FUNCTION "CENTR. 6  LATERALE SX" : VOID
TITLE =
VERSION : 0.1

BEGIN
NETWORK
TITLE =LETTURA STATUS WORD DA DRIVE
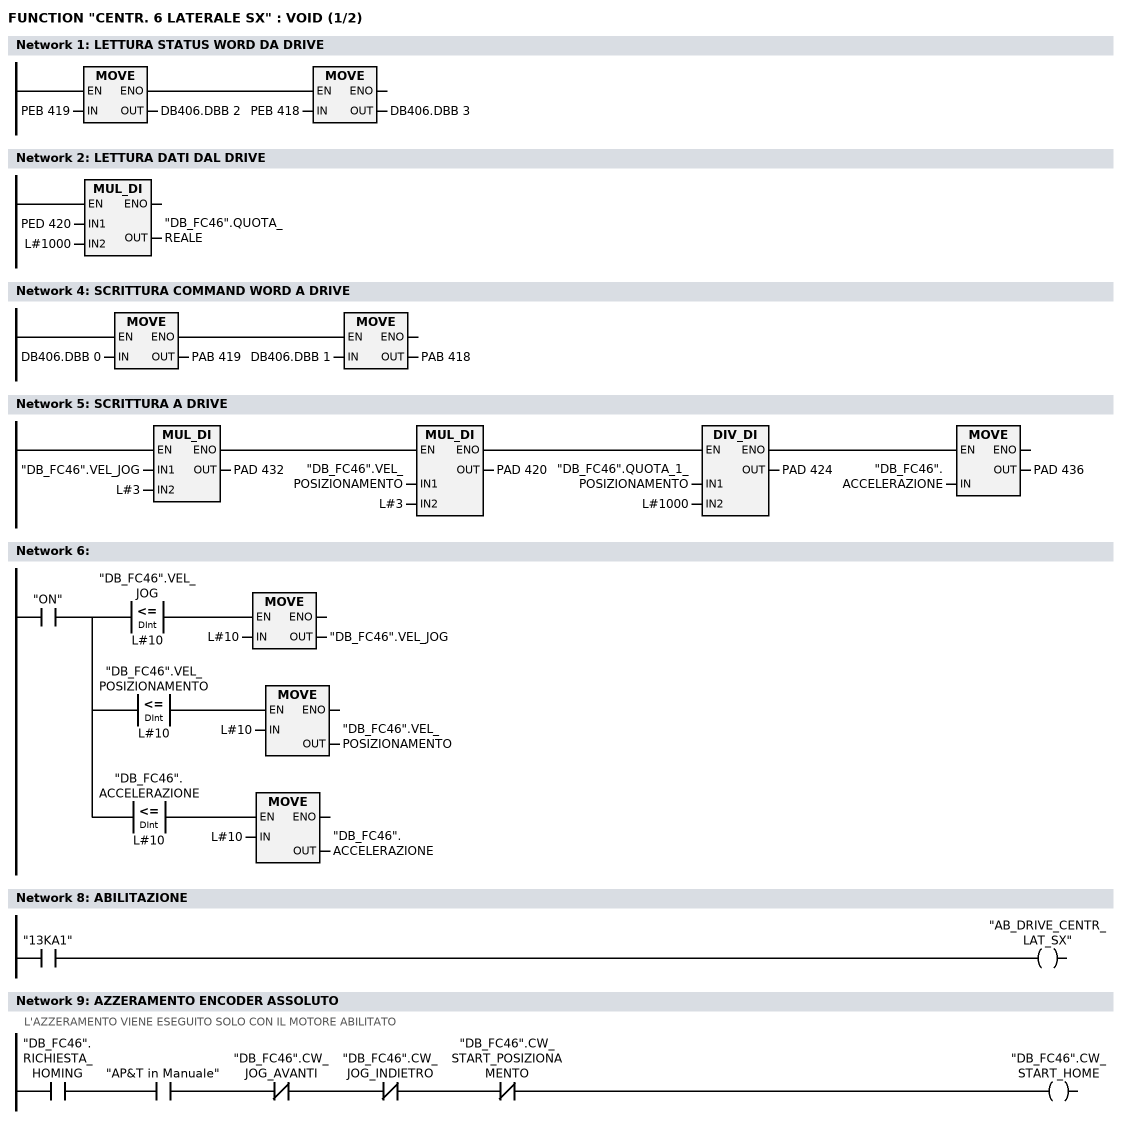
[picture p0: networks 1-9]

      U(    ;
      L     PEB  419;
      T     DB406.DBB    2;
      SET   ;
      SAVE  ;
      CLR   ;
      U     BIE;
      )     ;
      SPBNB _001;
      L     PEB  418;
      T     DB406.DBB    3;
_001: NOP   0;
NETWORK
TITLE =LETTURA DATI DAL DRIVE

      L     PED  420;
      L     L#1000;
      *D    ;
      T     "DB_FC46".QUOTA_REALE;
      NOP   0;
NETWORK
TITLE =

NETWORK
TITLE =SCRITTURA COMMAND WORD A DRIVE

      U(    ;
      L     DB406.DBB    0;
      T     PAB  419;
      SET   ;
      SAVE  ;
      CLR   ;
      U     BIE;
      )     ;
      SPBNB _002;
      L     DB406.DBB    1;
      T     PAB  418;
_002: NOP   0;
NETWORK
TITLE =SCRITTURA A DRIVE

      U(    ;
      U(    ;
      U(    ;
      L     "DB_FC46".VEL_JOG;
      L     L#3;
      *D    ;
      T     PAD  432;
      UN    OV;
      SAVE  ;
      CLR   ;
      U     BIE;
      )     ;
      SPBNB _003;
      L     "DB_FC46".VEL_POSIZIONAMENTO;
      L     L#3;
      *D    ;
      T     PAD  420;
      UN    OV;
      SAVE  ;
      CLR   ;
_003: U     BIE;
      )     ;
      SPBNB _004;
      L     "DB_FC46".QUOTA_1_POSIZIONAMENTO;
      L     L#1000;
      /D    ;
      T     PAD  424;
      UN    OV;
      SAVE  ;
      CLR   ;
_004: U     BIE;
      )     ;
      SPBNB _005;
      L     "DB_FC46".ACCELERAZIONE;
      T     PAD  436;
_005: NOP   0;
NETWORK
TITLE =

      U     "ON";
      =     L      0.0;
      U     L      0.0;
      U(    ;
      L     "DB_FC46".VEL_JOG;
      L     L#10;
      <=D   ;
      )     ;
      SPBNB _006;
      L     L#10;
      T     "DB_FC46".VEL_JOG;
_006: NOP   0;
      U     L      0.0;
      U(    ;
      L     "DB_FC46".VEL_POSIZIONAMENTO;
      L     L#10;
      <=D   ;
      )     ;
      SPBNB _007;
      L     L#10;
      T     "DB_FC46".VEL_POSIZIONAMENTO;
_007: NOP   0;
      U     L      0.0;
      U(    ;
      L     "DB_FC46".ACCELERAZIONE;
      L     L#10;
      <=D   ;
      )     ;
      SPBNB _008;
      L     L#10;
      T     "DB_FC46".ACCELERAZIONE;
_008: NOP   0;
NETWORK
TITLE =

NETWORK
TITLE =ABILITAZIONE

      U     "13KA1";
      =     "AB_DRIVE_CENTR_LAT_SX";
NETWORK
TITLE =AZZERAMENTO ENCODER ASSOLUTO
//L'AZZERAMENTO VIENE ESEGUITO SOLO CON IL MOTORE ABILITATO
      U     "DB_FC46".RICHIESTA_HOMING;
      U     "AP&T in Manuale";
      UN    "DB_FC46".CW_JOG_AVANTI;
      UN    "DB_FC46".CW_JOG_INDIETRO;
      UN    "DB_FC46".CW_START_POSIZIONAMENTO;
      =     "DB_FC46".CW_START_HOME;
NETWORK
TITLE =COMANDI DI JOG
//N.B. VERIFICARE QUOTE EXTRACORSA SOFTWARE
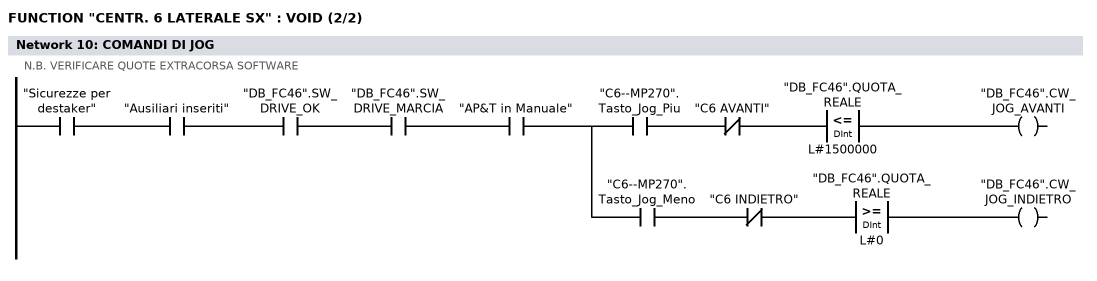
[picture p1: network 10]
      U     "Sicurezze per destaker";
      U     "Ausiliari inseriti";
      U     "DB_FC46".SW_DRIVE_OK;
      U     "DB_FC46".SW_DRIVE_MARCIA;
      U     "AP&T in Manuale";
      =     L      0.0;
      U     L      0.0;
      U     "C6--MP270".Tasto_Jog_Piu;
      UN    "C6 AVANTI";
      U(    ;
      L     "DB_FC46".QUOTA_REALE;
      L     L#1500000;
      <=D   ;
      )     ;
      =     "DB_FC46".CW_JOG_AVANTI;
      U     L      0.0;
      U     "C6--MP270".Tasto_Jog_Meno;
      UN    "C6 INDIETRO";
      U(    ;
      L     "DB_FC46".QUOTA_REALE;
      L     L#0;
      >=D   ;
      )     ;
      =     "DB_FC46".CW_JOG_INDIETRO;
NETWORK
TITLE =Centratore 6: Posizioni

      U     "ON";
      =     L      0.0;
      U     L      0.0;
      U(    ;
      L     "DB_FC46".QUOTA_REALE;
      L     L#100;
      <=D   ;
      )     ;
      U(    ;
      L     "DB_FC46".QUOTA_REALE;
      L     L#-100;
      >=D   ;
      )     ;
      =     "C6: Asse in pos.0";
      U(    ;
      U(    ;
      U     L      0.0;
      SPBNB _009;
      L     "MATRICOLA ATTUALE".C6_Posizione_1;
      L     L#100;
      -D    ;
      T     "CONFRONTI CENTRATORI".C6_Pos_1_Min;
      UN    OV;
      SAVE  ;
      CLR   ;
_009: U     BIE;
      )     ;
      SPBNB _00a;
      L     "MATRICOLA ATTUALE".C6_Posizione_1;
      L     L#200;
      +D    ;
      T     "CONFRONTI CENTRATORI".C6_Pos_1_Max;
      UN    OV;
      SAVE  ;
      CLR   ;
_00a: U     BIE;
      )     ;
      U(    ;
      L     "DB_FC46".QUOTA_REALE;
      L     "CONFRONTI CENTRATORI".C6_Pos_1_Min;
      >=D   ;
      )     ;
      U(    ;
      L     "DB_FC46".QUOTA_REALE;
      L     "CONFRONTI CENTRATORI".C6_Pos_1_Max;
      <=D   ;
      )     ;
      =     "C6: Asse in pos.1";
      U(    ;
      U(    ;
      U     L      0.0;
      SPBNB _00b;
      L     "MATRICOLA ATTUALE".C6_Posizione_2;
      L     L#100;
      -D    ;
      T     "CONFRONTI CENTRATORI".C6_Pos_2_Min;
      UN    OV;
      SAVE  ;
      CLR   ;
_00b: U     BIE;
      )     ;
      SPBNB _00c;
      L     "MATRICOLA ATTUALE".C6_Posizione_2;
      L     L#50000;
      +D    ;
      T     "CONFRONTI CENTRATORI".C6_Pos_2_Max;
      UN    OV;
      SAVE  ;
      CLR   ;
_00c: U     BIE;
      )     ;
      U(    ;
      L     "DB_FC46".QUOTA_REALE;
      L     "CONFRONTI CENTRATORI".C6_Pos_2_Min;
      >=D   ;
      )     ;
      UN    "C6: Asse in pos.3";
      UN    "C6: Asse in pos.4";
      =     "C6: Asse in pos.2";
      U(    ;
      U(    ;
      U     L      0.0;
      SPBNB _00d;
      L     "MATRICOLA ATTUALE".C6_Posizione_3;
      L     L#100;
      -D    ;
      T     "CONFRONTI CENTRATORI".C6_Pos_3_Min;
      UN    OV;
      SAVE  ;
      CLR   ;
_00d: U     BIE;
      )     ;
      SPBNB _00e;
      L     "MATRICOLA ATTUALE".C6_Posizione_3;
      L     L#50000;
      +D    ;
      T     "CONFRONTI CENTRATORI".C6_Pos_3_Max;
      UN    OV;
      SAVE  ;
      CLR   ;
_00e: U     BIE;
      )     ;
      U(    ;
      L     "DB_FC46".QUOTA_REALE;
      L     "CONFRONTI CENTRATORI".C6_Pos_3_Min;
      >=D   ;
      )     ;
      UN    "C6: Asse in pos.4";
      =     "C6: Asse in pos.3";
      U(    ;
      U(    ;
      U     L      0.0;
      SPBNB _00f;
      L     "MATRICOLA ATTUALE".C6_Posizione_4;
      L     L#100;
      -D    ;
      T     "CONFRONTI CENTRATORI".C6_Pos_4_Min;
      UN    OV;
      SAVE  ;
      CLR   ;
_00f: U     BIE;
      )     ;
      SPBNB _010;
      L     "MATRICOLA ATTUALE".C6_Posizione_4;
      L     L#100;
      +D    ;
      T     "CONFRONTI CENTRATORI".C6_Pos_4_Max;
      UN    OV;
      SAVE  ;
      CLR   ;
_010: U     BIE;
      )     ;
      U(    ;
      L     "DB_FC46".QUOTA_REALE;
      L     "CONFRONTI CENTRATORI".C6_Pos_4_Min;
      >=D   ;
      )     ;
      U(    ;
      L     "DB_FC46".QUOTA_REALE;
      L     "CONFRONTI CENTRATORI".C6_Pos_4_Max;
      <=D   ;
      )     ;
      =     "C6: Asse in pos.4";
NETWORK
TITLE =Centratore 6: consenso abilitazione passi
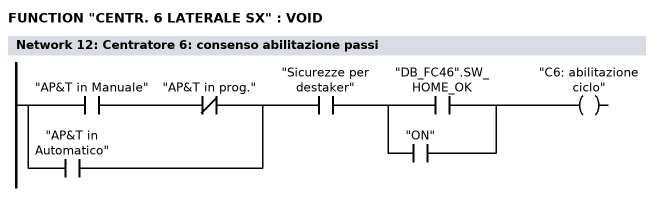
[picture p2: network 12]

      U(    ;
      U     "AP&T in Manuale";
      UN    "AP&T in prog.";
      O     "AP&T in Automatico";
      )     ;
      U     "Sicurezze per destaker";
      U(    ;
      O     "DB_FC46".SW_HOME_OK;
      O     "ON";
      )     ;
      =     "C6: abilitazione ciclo";
NETWORK
TITLE =Centratore 6: comando avvicinamento  (centraggi aperti)

      U(    ;
      U(    ;
      O     "Comando apre centraggi";
      O     "C6--MP270".Tasto_Indietro;
      O     ;
      U     "Apertura centratori";
      U(    ;
      O     "Centratori a riposo";
      O     "Centratori tutti chiusi";
      )     ;
      )     ;
      UN    "C6: Asse in pos.1";
      UN    "C6: comando arrivo";
      UN    "C6: comando a riposo";
      U     "C6: abilitazione ciclo";
      L     S5T#100MS;
      SE    T    197;
      NOP   0;
      NOP   0;
      NOP   0;
      U     T    197;
      )     ;
      S     "C6: comando avvicinam";
      U(    ;
      O     "C6: Asse in pos.1";
      O(    ;
      U(    ;
      O     "Ripristino centratori";
      O     "Comando riposo centraggi";
      O     "C6--MP270".Tasto_Riposo;
      )     ;
      FP    "C6: one shot 1";
      )     ;
      )     ;
      R     "C6: comando avvicinam";
      NOP   0;
NETWORK
TITLE =Centratore 6: comando arrivo (centraggi chiusi)

      U(    ;
      U(    ;
      O     "Comando chiude centraggi";
      O     "C6--MP270".Tasto_Avanti;
      O     ;
      U     "Chiusura centratori";
      U(    ;
      O     "Centratori tutti aperti";
      O     "Centratori a riposo";
      )     ;
      )     ;
      UN    "C6: Asse in pos.4";
      UN    "C6: comando avvicinam";
      UN    "C6: comando a riposo";
      U     "C6: abilitazione ciclo";
      L     S5T#100MS;
      SE    T    198;
      NOP   0;
      NOP   0;
      NOP   0;
      U     T    198;
      )     ;
      S     "C6: comando arrivo";
      U(    ;
      O     "C6: Asse in pos.4";
      O(    ;
      U(    ;
      O     "Ripristino centratori";
      O     "Comando riposo centraggi";
      O     "C6--MP270".Tasto_Riposo;
      )     ;
      FP    "C6: one shot 2";
      )     ;
      )     ;
      R     "C6: comando arrivo";
      NOP   0;
NETWORK
TITLE =Centratore 6: comando automatico centraggi a riposo

      U(    ;
      U(    ;
      O     "Comando riposo centraggi";
      O     "C6--MP270".Tasto_Riposo;
      )     ;
      UN    "C6: Asse in pos.0";
      UN    "C6: comando avvicinam";
      UN    "C6: comando arrivo";
      U     "C6: abilitazione ciclo";
      L     S5T#100MS;
      SE    T    199;
      NOP   0;
      NOP   0;
      NOP   0;
      U     T    199;
      )     ;
      S     "C6: comando a riposo";
      U(    ;
      O     "C6: Asse in pos.0";
      O(    ;
      U     "Ripristino centratori";
      FP    "C6: one shot 3";
      )     ;
      )     ;
      R     "C6: comando a riposo";
      NOP   0;
NETWORK
TITLE =Centratore 6: quote impostate per posizioni

      U     "ON";
      =     L      0.0;
      U(    ;
      U(    ;
      U     L      0.0;
      U     "C6: comando a riposo";
      UN    "C6: Asse in pos.0";
      SPBNB _011;
      L     0;
      T     "DB_FC46".QUOTA_1_POSIZIONAMENTO;
      SET   ;
      SAVE  ;
      CLR   ;
_011: U     BIE;
      )     ;
      SPBNB _012;
      L     L#150;
      T     "DB_FC46".VEL_POSIZIONAMENTO;
      SET   ;
      SAVE  ;
      CLR   ;
_012: U     BIE;
      )     ;
      SPBNB _013;
      L     L#1000;
      T     "DB_FC46".ACCELERAZIONE;
      SET   ;
      SAVE  ;
      CLR   ;
_013: U     BIE;
      =     "C6: Quote pronte pos.0";
      U(    ;
      U(    ;
      U     L      0.0;
      U     "C6: comando avvicinam";
      UN    "C6: Asse in pos.1";
      SPBNB _014;
      L     "MATRICOLA ATTUALE".C6_Posizione_1;
      T     "DB_FC46".QUOTA_1_POSIZIONAMENTO;
      SET   ;
      SAVE  ;
      CLR   ;
_014: U     BIE;
      )     ;
      SPBNB _015;
      L     "MATRICOLA ATTUALE".C6_Velocita_1;
      T     "DB_FC46".VEL_POSIZIONAMENTO;
      SET   ;
      SAVE  ;
      CLR   ;
_015: U     BIE;
      )     ;
      SPBNB _016;
      L     "MATRICOLA ATTUALE".C6_Accell_1;
      T     "DB_FC46".ACCELERAZIONE;
      SET   ;
      SAVE  ;
      CLR   ;
_016: U     BIE;
      =     "C6: Quote pronte pos.1";
      U     L      0.0;
      U     "C6: comando arrivo";
      =     L      0.1;
      U(    ;
      U(    ;
      U     L      0.1;
      UN    "C6: Asse in pos.2";
      SPBNB _017;
      L     "MATRICOLA ATTUALE".C6_Posizione_4;
      T     "DB_FC46".QUOTA_1_POSIZIONAMENTO;
      SET   ;
      SAVE  ;
      CLR   ;
_017: U     BIE;
      )     ;
      SPBNB _018;
      L     "MATRICOLA ATTUALE".C6_Velocita_2;
      T     "DB_FC46".VEL_POSIZIONAMENTO;
      SET   ;
      SAVE  ;
      CLR   ;
_018: U     BIE;
      )     ;
      SPBNB _019;
      L     "MATRICOLA ATTUALE".C6_Accell_2;
      T     "DB_FC46".ACCELERAZIONE;
      SET   ;
      SAVE  ;
      CLR   ;
_019: U     BIE;
      S     "C6: Quote pronte pos.2";
      U     L      0.1;
      U     "C6: Quote pronte pos.2";
      UN    "C6: Reset start pos.2";
      L     S5T#1S;
      SE    "C6: ritardo P2";
      NOP   0;
      NOP   0;
      NOP   0;
      U     "C6: ritardo P2";
      S     "C6: Reset start pos.2";
      R     "C6: Quote pronte pos.2";
      U     L      0.0;
      U     "C6: comando arrivo";
      =     L      0.1;
      U(    ;
      U(    ;
      U(    ;
      U     L      0.1;
      U     "C6: Asse in pos.2";
      UN    "C6: Asse in pos.3";
      SPBNB _01a;
      L     "MATRICOLA ATTUALE".C6_Posizione_4;
      T     "DB_FC46".QUOTA_1_POSIZIONAMENTO;
      SET   ;
      SAVE  ;
      CLR   ;
_01a: U     BIE;
      )     ;
      SPBNB _01b;
      L     "MATRICOLA ATTUALE".C6_Velocita_3;
      T     "DB_FC46".VEL_POSIZIONAMENTO;
      SET   ;
      SAVE  ;
      CLR   ;
_01b: U     BIE;
      )     ;
      SPBNB _01c;
      L     "MATRICOLA ATTUALE".C6_Accell_3;
      T     "DB_FC46".ACCELERAZIONE;
      SET   ;
      SAVE  ;
      CLR   ;
_01c: U     BIE;
      )     ;
      U     "C6: Reset start pos.2";
      S     "C6: Quote pronte pos.3";
      R     "C6: Reset start pos.2";
      U     L      0.1;
      U     "C6: Quote pronte pos.3";
      L     S5T#500MS;
      SE    "C6: ritardo P3";
      NOP   0;
      NOP   0;
      NOP   0;
      U     "C6: ritardo P3";
      S     "C6: Reset start pos.3";
      R     "C6: Quote pronte pos.3";
      U     L      0.0;
      U     "C6: comando arrivo";
      =     L      0.1;
      U(    ;
      U(    ;
      U(    ;
      U     L      0.1;
      U     "C6: Asse in pos.3";
      UN    "C6: Asse in pos.4";
      SPBNB _01d;
      L     "MATRICOLA ATTUALE".C6_Posizione_4;
      T     "DB_FC46".QUOTA_1_POSIZIONAMENTO;
      SET   ;
      SAVE  ;
      CLR   ;
_01d: U     BIE;
      )     ;
      SPBNB _01e;
      L     "MATRICOLA ATTUALE".C6_Velocita_4;
      T     "DB_FC46".VEL_POSIZIONAMENTO;
      SET   ;
      SAVE  ;
      CLR   ;
_01e: U     BIE;
      )     ;
      SPBNB _01f;
      L     "MATRICOLA ATTUALE".C6_Accell_4;
      T     "DB_FC46".ACCELERAZIONE;
      SET   ;
      SAVE  ;
      CLR   ;
_01f: U     BIE;
      )     ;
      U     "C6: Reset start pos.3";
      S     "C6: Quote pronte pos.4";
      R     "C6: Reset start pos.3";
      U     L      0.1;
      U     "C6: Quote pronte pos.4";
      L     S5T#500MS;
      SE    "C6: ritardo P4";
      NOP   0;
      NOP   0;
      NOP   0;
      U     "C6: ritardo P4";
      S     "C6: Reset start pos.4";
      R     "C6: Quote pronte pos.4";
NETWORK
TITLE =Centratore 6: reset impostate
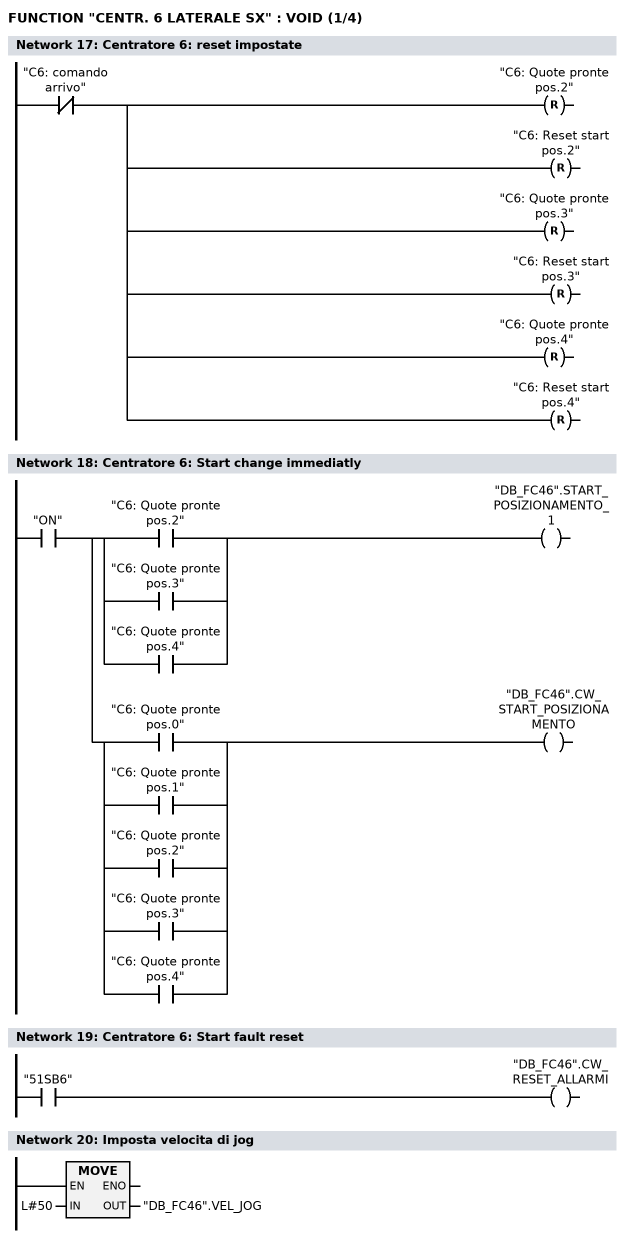
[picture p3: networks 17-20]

      UN    "C6: comando arrivo";
      R     "C6: Quote pronte pos.2";
      R     "C6: Reset start pos.2";
      R     "C6: Quote pronte pos.3";
      R     "C6: Reset start pos.3";
      R     "C6: Quote pronte pos.4";
      R     "C6: Reset start pos.4";
NETWORK
TITLE =Centratore 6: Start change immediatly

      U     "ON";
      =     L      0.0;
      U     L      0.0;
      U(    ;
      O     "C6: Quote pronte pos.2";
      O     "C6: Quote pronte pos.3";
      O     "C6: Quote pronte pos.4";
      )     ;
      =     "DB_FC46".START_POSIZIONAMENTO_1;
      U     L      0.0;
      U(    ;
      O     "C6: Quote pronte pos.0";
      O     "C6: Quote pronte pos.1";
      O     "C6: Quote pronte pos.2";
      O     "C6: Quote pronte pos.3";
      O     "C6: Quote pronte pos.4";
      )     ;
      =     "DB_FC46".CW_START_POSIZIONAMENTO;
NETWORK
TITLE =Centratore 6: Start fault reset

      U     "51SB6";
      =     "DB_FC46".CW_RESET_ALLARMI;
NETWORK
TITLE =Imposta velocita di jog

      L     L#50;
      T     "DB_FC46".VEL_JOG;
      NOP   0;
NETWORK
TITLE =Centratore 6: Drive Enable ok
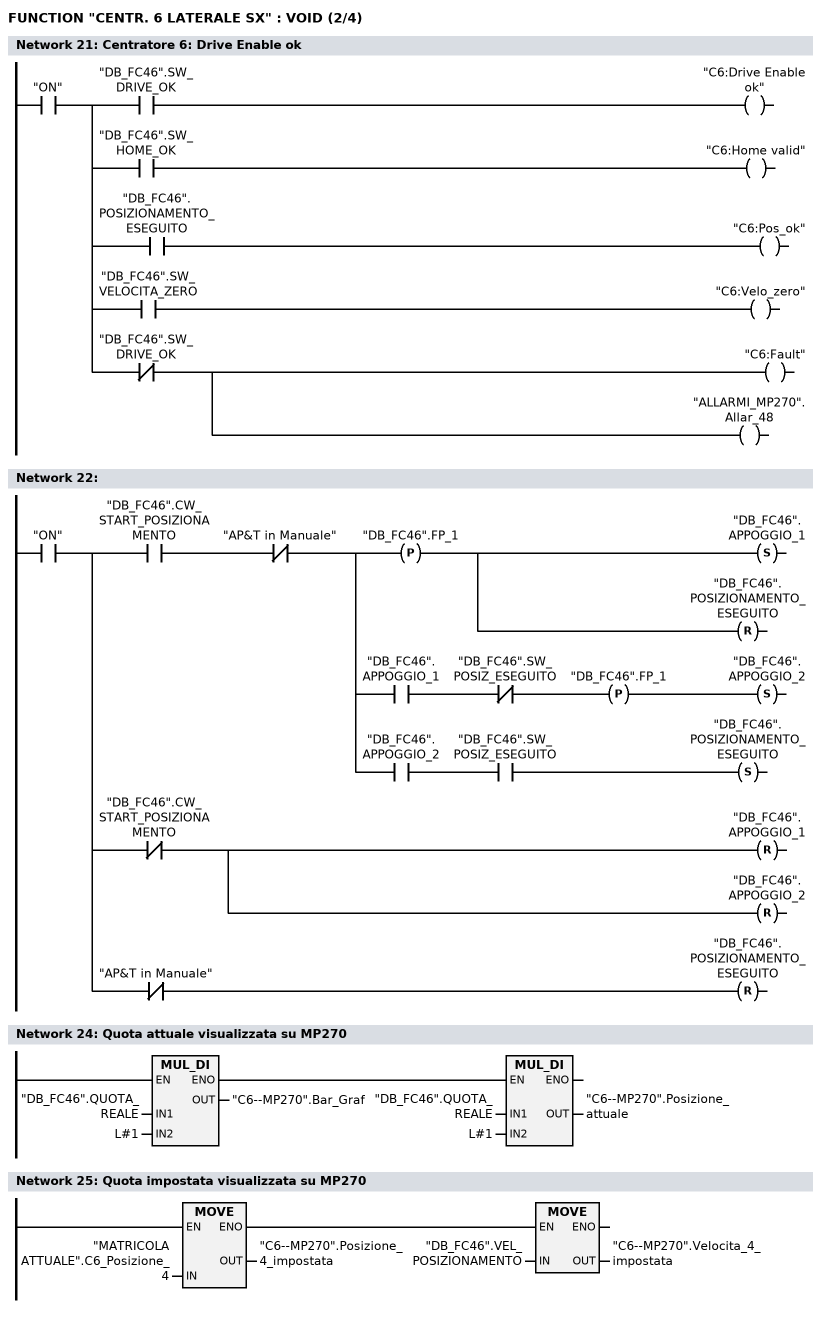
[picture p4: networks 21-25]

      U     "ON";
      =     L      0.0;
      U     L      0.0;
      U     "DB_FC46".SW_DRIVE_OK;
      =     "C6:Drive Enable ok";
      U     L      0.0;
      U     "DB_FC46".SW_HOME_OK;
      =     "C6:Home valid";
      U     L      0.0;
      U     "DB_FC46".POSIZIONAMENTO_ESEGUITO;
      =     "C6:Pos_ok";
      U     L      0.0;
      U     "DB_FC46".SW_VELOCITA_ZERO;
      =     "C6:Velo_zero";
      U     L      0.0;
      UN    "DB_FC46".SW_DRIVE_OK;
      =     "C6:Fault";
      =     "ALLARMI_MP270".Allar_48;
NETWORK
TITLE =

      U     "ON";
      =     L      0.0;
      U     L      0.0;
      U     "DB_FC46".CW_START_POSIZIONAMENTO;
      UN    "AP&T in Manuale";
      =     L      0.1;
      U     L      0.1;
      FP    "DB_FC46".FP_1;
      S     "DB_FC46".APPOGGIO_1;
      R     "DB_FC46".POSIZIONAMENTO_ESEGUITO;
      U     L      0.1;
      U     "DB_FC46".APPOGGIO_1;
      UN    "DB_FC46".SW_POSIZ_ESEGUITO;
      FP    "DB_FC46".FP_1;
      S     "DB_FC46".APPOGGIO_2;
      U     L      0.1;
      U     "DB_FC46".APPOGGIO_2;
      U     "DB_FC46".SW_POSIZ_ESEGUITO;
      S     "DB_FC46".POSIZIONAMENTO_ESEGUITO;
      U     L      0.0;
      UN    "DB_FC46".CW_START_POSIZIONAMENTO;
      R     "DB_FC46".APPOGGIO_1;
      R     "DB_FC46".APPOGGIO_2;
      U     L      0.0;
      UN    "AP&T in Manuale";
      R     "DB_FC46".POSIZIONAMENTO_ESEGUITO;
NETWORK
TITLE =

NETWORK
TITLE =Quota attuale visualizzata su MP270

      U(    ;
      L     "DB_FC46".QUOTA_REALE;
      L     L#1;
      *D    ;
      T     "C6--MP270".Bar_Graf;
      UN    OV;
      SAVE  ;
      CLR   ;
      U     BIE;
      )     ;
      SPBNB _020;
      L     "DB_FC46".QUOTA_REALE;
      L     L#1;
      *D    ;
      T     "C6--MP270".Posizione_attuale;
_020: NOP   0;
NETWORK
TITLE =Quota impostata visualizzata su MP270

      U(    ;
      L     "MATRICOLA ATTUALE".C6_Posizione_4;
      T     "C6--MP270".Posizione_4_impostata;
      SET   ;
      SAVE  ;
      CLR   ;
      U     BIE;
      )     ;
      SPBNB _021;
      L     "DB_FC46".VEL_POSIZIONAMENTO;
      T     "C6--MP270".Velocita_4_impostata;
_021: NOP   0;
NETWORK
TITLE =Visualizza FC su MP270
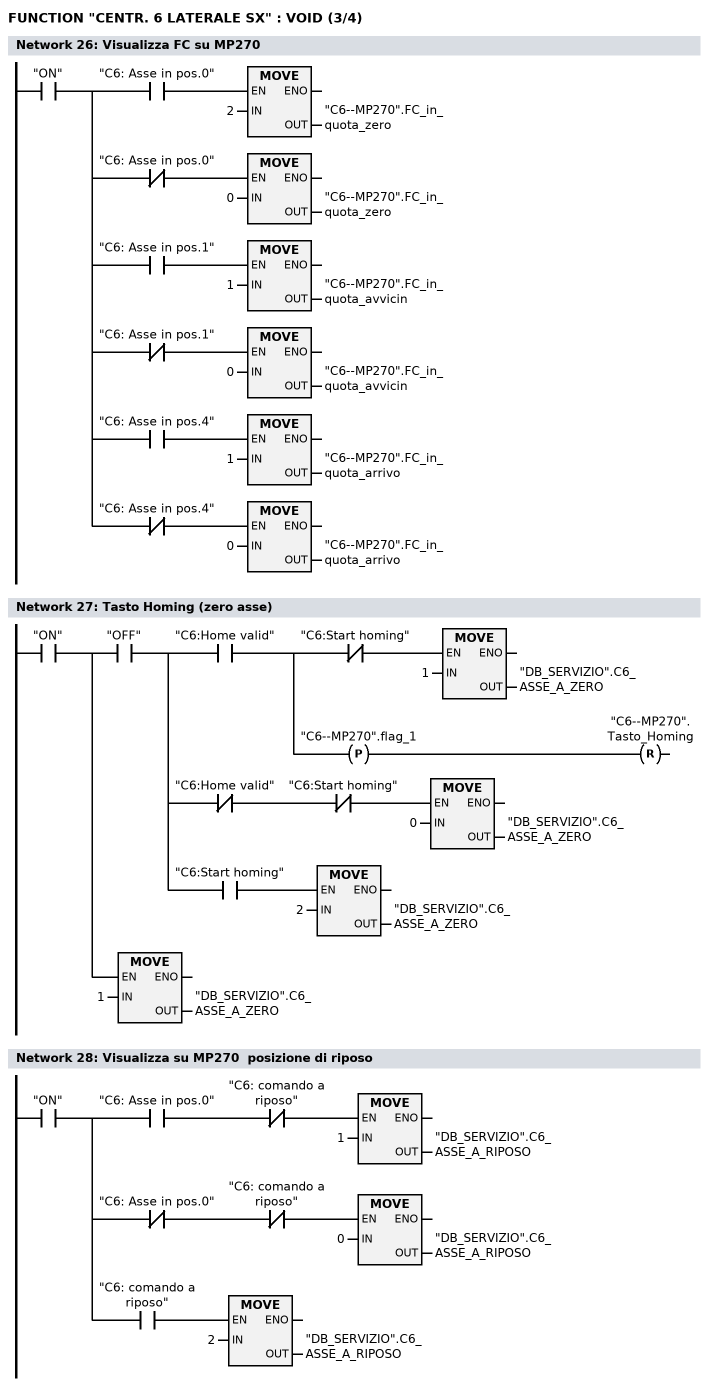
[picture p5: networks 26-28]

      U     "ON";
      =     L      0.0;
      U     L      0.0;
      U     "C6: Asse in pos.0";
      SPBNB _022;
      L     2;
      T     "C6--MP270".FC_in_quota_zero;
_022: NOP   0;
      U     L      0.0;
      UN    "C6: Asse in pos.0";
      SPBNB _023;
      L     0;
      T     "C6--MP270".FC_in_quota_zero;
_023: NOP   0;
      U     L      0.0;
      U     "C6: Asse in pos.1";
      SPBNB _024;
      L     1;
      T     "C6--MP270".FC_in_quota_avvicin;
_024: NOP   0;
      U     L      0.0;
      UN    "C6: Asse in pos.1";
      SPBNB _025;
      L     0;
      T     "C6--MP270".FC_in_quota_avvicin;
_025: NOP   0;
      U     L      0.0;
      U     "C6: Asse in pos.4";
      SPBNB _026;
      L     1;
      T     "C6--MP270".FC_in_quota_arrivo;
_026: NOP   0;
      U     L      0.0;
      UN    "C6: Asse in pos.4";
      SPBNB _027;
      L     0;
      T     "C6--MP270".FC_in_quota_arrivo;
_027: NOP   0;
NETWORK
TITLE =Tasto Homing (zero asse)

      U     "ON";
      =     L      0.0;
      U     L      0.0;
      U     "OFF";
      =     L      0.1;
      U     L      0.1;
      U     "C6:Home valid";
      =     L      0.2;
      U     L      0.2;
      UN    "C6:Start homing";
      SPBNB _028;
      L     1;
      T     "DB_SERVIZIO".C6_ASSE_A_ZERO;
_028: NOP   0;
      U     L      0.2;
      FP    "C6--MP270".flag_1;
      R     "C6--MP270".Tasto_Homing;
      U     L      0.1;
      UN    "C6:Home valid";
      UN    "C6:Start homing";
      SPBNB _029;
      L     0;
      T     "DB_SERVIZIO".C6_ASSE_A_ZERO;
_029: NOP   0;
      U     L      0.1;
      U     "C6:Start homing";
      SPBNB _02a;
      L     2;
      T     "DB_SERVIZIO".C6_ASSE_A_ZERO;
_02a: NOP   0;
      U     L      0.0;
      SPBNB _02b;
      L     1;
      T     "DB_SERVIZIO".C6_ASSE_A_ZERO;
_02b: NOP   0;
NETWORK
TITLE =Visualizza su MP270  posizione di riposo

      U     "ON";
      =     L      0.0;
      U     L      0.0;
      U     "C6: Asse in pos.0";
      UN    "C6: comando a riposo";
      SPBNB _02c;
      L     1;
      T     "DB_SERVIZIO".C6_ASSE_A_RIPOSO;
_02c: NOP   0;
      U     L      0.0;
      UN    "C6: Asse in pos.0";
      UN    "C6: comando a riposo";
      SPBNB _02d;
      L     0;
      T     "DB_SERVIZIO".C6_ASSE_A_RIPOSO;
_02d: NOP   0;
      U     L      0.0;
      U     "C6: comando a riposo";
      SPBNB _02e;
      L     2;
      T     "DB_SERVIZIO".C6_ASSE_A_RIPOSO;
_02e: NOP   0;
NETWORK
TITLE =Visualizza su MP270  posizione di avvicinamento
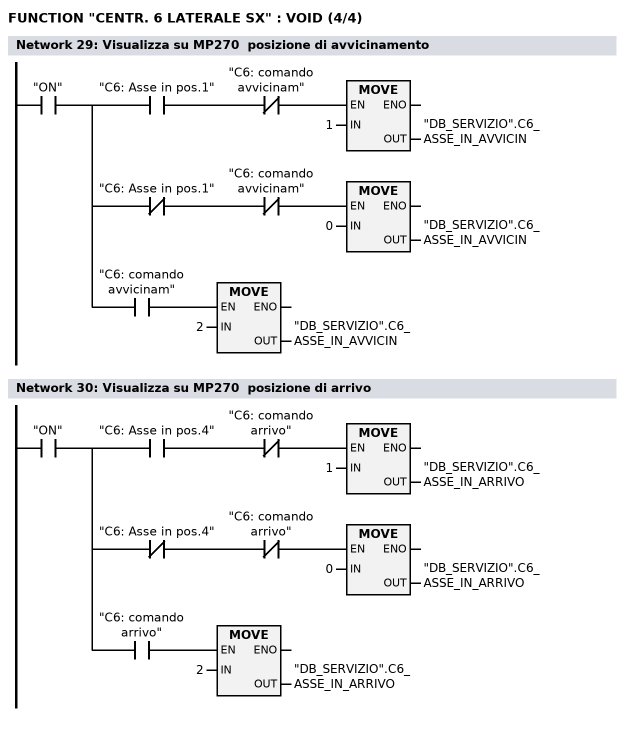
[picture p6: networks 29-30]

      U     "ON";
      =     L      0.0;
      U     L      0.0;
      U     "C6: Asse in pos.1";
      UN    "C6: comando avvicinam";
      SPBNB _02f;
      L     1;
      T     "DB_SERVIZIO".C6_ASSE_IN_AVVICIN;
_02f: NOP   0;
      U     L      0.0;
      UN    "C6: Asse in pos.1";
      UN    "C6: comando avvicinam";
      SPBNB _030;
      L     0;
      T     "DB_SERVIZIO".C6_ASSE_IN_AVVICIN;
_030: NOP   0;
      U     L      0.0;
      U     "C6: comando avvicinam";
      SPBNB _031;
      L     2;
      T     "DB_SERVIZIO".C6_ASSE_IN_AVVICIN;
_031: NOP   0;
NETWORK
TITLE =Visualizza su MP270  posizione di arrivo

      U     "ON";
      =     L      0.0;
      U     L      0.0;
      U     "C6: Asse in pos.4";
      UN    "C6: comando arrivo";
      SPBNB _032;
      L     1;
      T     "DB_SERVIZIO".C6_ASSE_IN_ARRIVO;
_032: NOP   0;
      U     L      0.0;
      UN    "C6: Asse in pos.4";
      UN    "C6: comando arrivo";
      SPBNB _033;
      L     0;
      T     "DB_SERVIZIO".C6_ASSE_IN_ARRIVO;
_033: NOP   0;
      U     L      0.0;
      U     "C6: comando arrivo";
      SPBNB _034;
      L     2;
      T     "DB_SERVIZIO".C6_ASSE_IN_ARRIVO;
_034: NOP   0;
END_FUNCTION

